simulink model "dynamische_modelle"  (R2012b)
settings: Solver=ode45  StartTime=0.0  StopTime=10.0  RelTol=1e-3
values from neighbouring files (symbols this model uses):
  f = FG    (= 500)    [coulomb_5.m]    (also in dry_friction_1.m; feder_masse_1.m = logspace(e1,e2,5000); feder_masse_11.m = logspace(e1,e2,5000); feder_masse_12.m = logspace(e1,e2,5000))
  FG = 500    [coulomb_1.m]    (also in coulomb_10.m = 10; coulomb_11.m = 10; coulomb_2.m; coulomb_3.m)
  FH = 12    [coulomb_10.m]    (also in coulomb_11.m; coulomb_3.m = 600; coulomb_4.m = 600; position_reg_1.m = 3.956)
  sigma_0 = 5000    [position_reg_1.m]    (also in position_reg_2.m; slip_stick_21.m = 10000; slip_stick_s_12.m = 10000; tilger_gleitreib2.m = 1000)
  sigma_1 = sqrt(sigma_0)    [position_reg_1.m]    (also in position_reg_2.m; slip_stick_21.m = sqrt(1e5); slip_stick_s_12.m = sqrt(1e5); tilger_gleitreib2.m)
  sigma_2 = 0    [position_reg_1.m]    (also in position_reg_2.m; slip_stick_21.m; slip_stick_s_12.m; tilger_gleitreib2.m)
  vs = 0.05    [position_reg_1.m]    (also in position_reg_2.m; slip_stick_21.m; slip_stick_3.m = 0.01; slip_stick_31.m)

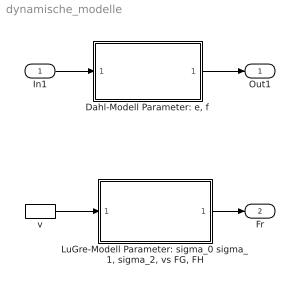
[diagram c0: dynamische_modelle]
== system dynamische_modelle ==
  In1 : Inport
  "Dahl-Modell Parameter: e, f" : Subsystem
  "LuGre-Modell Parameter: sigma_0 sigma_1, sigma_2, vs FG, FH" : Subsystem
  v : InportShadow
  Out1 : Outport
  Fr : Outport  Port=2
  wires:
  In1/1 -> "Dahl-Modell Parameter: e, f"/1(v)
  "Dahl-Modell Parameter: e, f"/1(Fr) -> Out1/1
  v/1 -> "LuGre-Modell Parameter: sigma_0 sigma_1, sigma_2, vs FG, FH"/1(v)
  "LuGre-Modell Parameter: sigma_0 sigma_1, sigma_2, vs FG, FH"/1(Fr) -> Fr/1

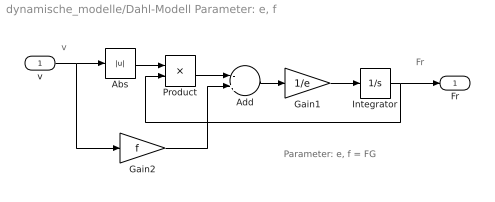
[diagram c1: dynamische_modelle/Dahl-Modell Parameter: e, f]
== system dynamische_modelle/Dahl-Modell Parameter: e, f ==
  note: Parameter: e, f = FG
  note: Fr
  note: v
  v : Inport
  Abs : Abs
  Add : Sum  Inputs=-+
  Gain1 : Gain  Gain=1/e
  Gain2 : Gain  Gain=f
  Integrator : Integrator
  Product : Product
  Fr : Outport
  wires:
  Gain1/1 -> Integrator/1
  Gain2/1 -> Add/2
  Product/1 -> Add/1
  v/1 -> Gain2/1, Abs/1
  Add/1 -> Gain1/1
  Abs/1 -> Product/1
  Integrator/1 -> Fr/1, Product/2

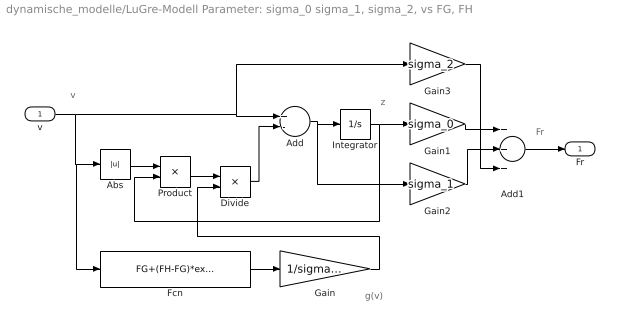
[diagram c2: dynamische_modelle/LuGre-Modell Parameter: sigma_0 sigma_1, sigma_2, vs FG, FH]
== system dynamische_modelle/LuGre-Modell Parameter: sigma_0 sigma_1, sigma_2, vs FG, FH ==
  note: Fr
  note: v
  note: g(v)
  note: z
  v : Inport
  Abs : Abs
  Add : Sum  Inputs=+-
  Add1 : Sum  Inputs=+++
  Divide : Product  Inputs=*/
  Fcn : Fcn  Expr=FG+(FH-FG)*exp(-(u/vs)^2)
  Gain : Gain  Gain=1/sigma_0
  Gain1 : Gain  Gain=sigma_0
  Gain2 : Gain  Gain=sigma_1
  Gain3 : Gain  Gain=sigma_2
  Integrator : Integrator
  Product : Product
  Fr : Outport
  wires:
  v/1 -> Gain3/1, Add/1, Fcn/1, Abs/1
  Integrator/1 -> Gain1/1, Product/2
  Add/1 -> Gain2/1, Integrator/1
  Gain2/1 -> Add1/2
  Abs/1 -> Product/1
  Divide/1 -> Add/2
  Gain1/1 -> Add1/1
  Add1/1 -> Fr/1
  Gain3/1 -> Add1/3
  Fcn/1 -> Gain/1
  Gain/1 -> Divide/2
  Product/1 -> Divide/1
